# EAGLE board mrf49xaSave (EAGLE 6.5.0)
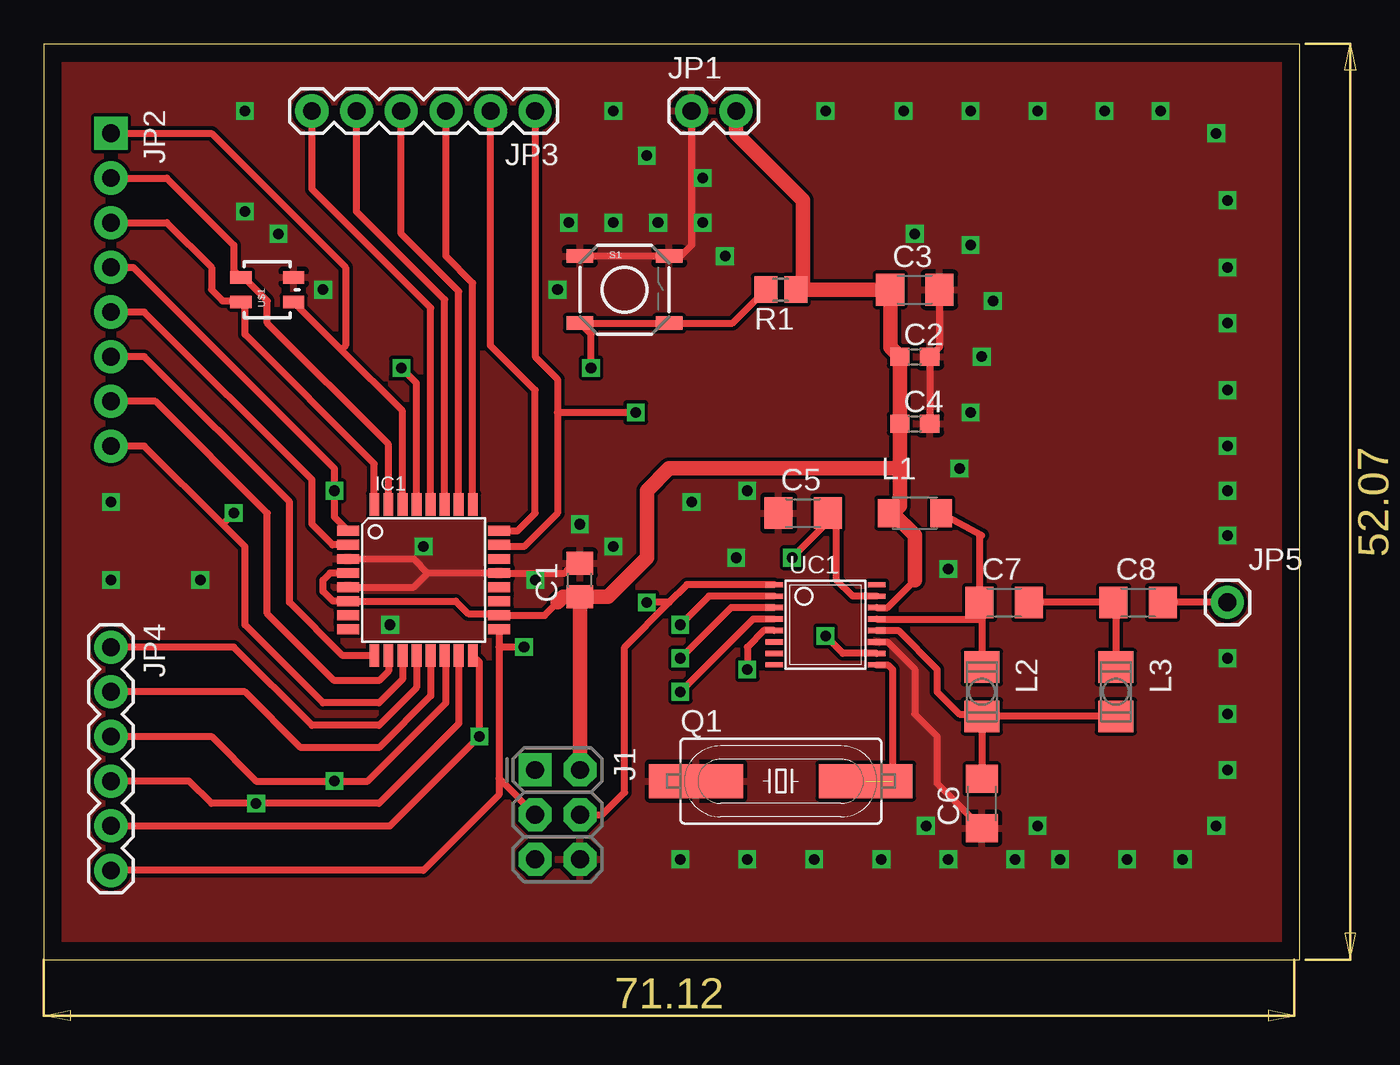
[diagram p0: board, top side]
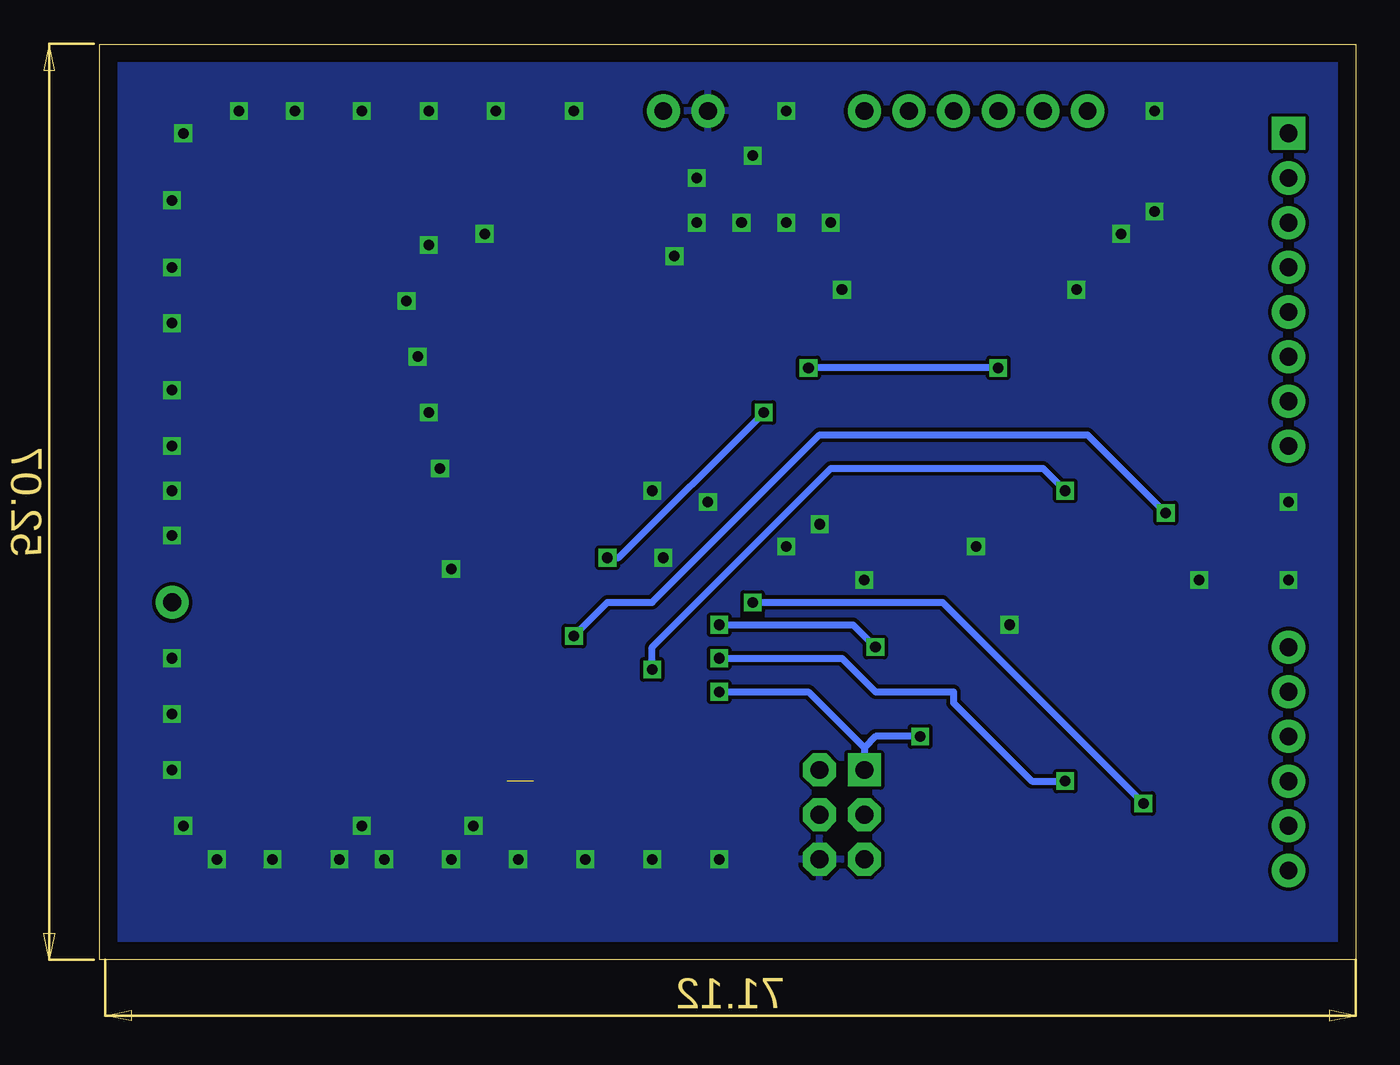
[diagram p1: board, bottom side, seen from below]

Size 74.59 x 55.55 mm. Coordinates in mm from the lower left corner, seen from the top.
Outline: 0,3.48 71.42,3.48 71.42,55.54 0,55.54 0,3.48
Copper layers (1*16): Top 0.035mm / dielectric 1.5mm / Bottom 0.035mm
Design rules "default": minimum track width 10mil, minimum drill 24mil, track to track 8mil, track to pad 8mil, pad to pad 8mil, via to via 8mil, smd to smd 8mil, copper to edge 40mil, drill to drill 8mil, minimum pad ring 10mil, minimum via ring 8mil, stop-mask expansion 4mil, vias tented up to drill 0mil, thermal gap 10mil

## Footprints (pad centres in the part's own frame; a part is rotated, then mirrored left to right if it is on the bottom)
C0805 = smd 1.3 x 1.5: 1 -0.95,0; 2 0.95,0
C0603 = smd 1.1 x 1: 1 -0.85,0; 2 0.85,0
C1206 = smd 1.6 x 1.8: 1 -1.4,0; 2 1.4,0
TQFP32-08 = smd 1.27 x 0.559: 1 -4.293,2.8; 2 -4.293,2; 3 -4.293,1.2; 4 -4.293,0.4; 5 -4.293,-0.4; 6 -4.293,-1.2; 7 -4.293,-2; 8 -4.293,-2.8; 17 4.293,-2.8; 18 4.293,-2; 19 4.293,-1.2; 20 4.293,-0.4; 21 4.293,0.4; 22 4.293,1.2; 23 4.293,2; 24 4.293,2.8 | smd 0.559 x 1.27: 9 -2.8,-4.293; 10 -2,-4.293; 11 -1.2,-4.293; 12 -0.4,-4.293; 13 0.4,-4.293; 14 1.2,-4.293; 15 2,-4.293; 16 2.8,-4.293; 25 2.8,4.293; 26 2,4.293; 27 1.2,4.293; 28 0.4,4.293; 29 -0.4,4.293; 30 -1.2,4.293; 31 -2,4.293; 32 -2.8,4.293
2X3-NS = drill 1.016 pad 1.88 square: 1 -2.54,-1.27 | drill 1.016 pad 1.88 octagon: 2 -2.54,1.27; 3 0,-1.27; 4 0,1.27; 5 2.54,-1.27; 6 2.54,1.27
1X02 = drill 1.016 pad 1.88: 1 0,0; 2 2.54,0
1X08_PIN1_NO_SILK = drill 1.016 pad 1.88 square: 1 0,0 | drill 1.016 pad 1.88: 2 2.54,0; 3 5.08,0; 4 7.62,0; 5 10.16,0; 6 12.7,0; 7 15.24,0; 8 17.78,0
1X06 = drill 1.016 pad 1.88: 1 0,0; 2 2.54,0; 3 5.08,0; 4 7.62,0; 5 10.16,0; 6 12.7,0
1X01 = drill 1.016 pad 1.88: 1 0,0
L3216C = smd 1.2 x 1.6: 1 -1.5,0; 2 1.5,0
L3225P = smd 1.8 x 2: 1 -1.4,0; 2 1.4,0
HC49UP = smd 5.334 x 1.93: 1 -4.826,0; 2 4.826,0
R2012 = smd 1.3 x 1.5: 1 -0.85,0; 2 0.85,0
TACTILE_SWITCH_SMD = smd 1.524 x 0.762: 1 -2.54,1.905; 2 2.54,1.905; 3 -2.54,-1.905; 4 2.54,-1.905
LED-TRICOLOR-SMD = smd 0.7 x 1.2: A 0.7,-1.5; B 0.7,1.5; G -0.7,1.5; R -0.7,-1.5
TSSOP16 = smd 0.305 x 0.991: 1 -2.275,-2.918; 2 -1.625,-2.918; 3 -0.975,-2.918; 4 -0.325,-2.918; 5 0.325,-2.918; 6 0.975,-2.918; 7 1.625,-2.918; 8 2.275,-2.918; 9 2.275,2.918; 10 1.625,2.918; 11 0.975,2.918; 12 0.325,2.918; 13 -0.325,2.918; 14 -0.975,2.918; 15 -1.625,2.918; 16 -2.275,2.918

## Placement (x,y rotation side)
C1  100nF  [C0805]  30.48,25.07 90 top
C2  0.01uF  [C0603]  49.53,37.77 0 top
C3  2.2uF  [C1206]  49.53,41.58 0 top
C4  47pF  [C0603]  49.53,33.95 0 top
C5  1000pF  [C1206]  43.18,28.88 0 top
C6  2.7pF  [C1206]  53.34,12.37 90 top
C7  1.2pF  [C1206]  54.61,23.79 0 top
C8  27pF  [C1206]  62.23,23.79 0 top
IC1  MEGA48/88/168-AU  [TQFP32-08]  21.59,25.07 0 top
J1  AVR_SPI_PRG_6NS  [2X3-NS]  29.21,11.73 270 top
JP1  M02PTH  [1X02]  36.83,51.73 0 top
JP2  [1X08_PIN1_NO_SILK]  3.81,50.47 270 top
JP3  [1X06]  27.94,51.73 180 top
JP4  [1X06]  3.81,21.25 270 top
JP5  M01PTH  [1X01]  67.31,23.79 0 top
L1  100nH  [L3216C]  49.53,28.88 0 top
L2  8.2nH  [L3225P]  53.34,18.71 270 top
L3  22nH  [L3225P]  60.96,18.71 270 top
Q1  10MHz  [HC49UP]  41.91,13.64 0 top
R1  10K  [R2012]  41.91,41.58 180 top
S1  [TACTILE_SWITCH_SMD]  33.02,41.58 0 top
U$1  LED-TRICOLOR  [LED-TRICOLOR-SMD]  12.7,41.58 90 top
UC1  MRF49XATSSOP163  [TSSOP16]  44.45,22.53 270 top

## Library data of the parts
C1-C8 L1-L3 = rcl
IC1 = avr-6
J1 JP1-JP5 = SparkFun-Connectors
Q1 = SparkFun
R1 = resistor
S1 = SparkFun-Electromechanical; PROD_ID: SWCH-08247
U$1 = SparkFun-LED
UC1 = nicolas

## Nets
+3V3: C1.1 C2.1 C3.1 C4.1 IC1.4 IC1.6 IC1.18 J1.2 JP1.2 L1.1 R1.1 UC1.14
BLUE: IC1.31 JP2.2 U$1.B
CS: IC1.14 JP4.3 UC1.3
GND: C1.2 C2.2 C3.2 C4.2 C5.1 C6.1 IC1.3 IC1.5 IC1.21 J1.6 JP1.1 Q1.1 S1.1 S1.2 U$1.A UC1.11
GRN: IC1.32 JP2.3 U$1.G
IRQ: IC1.1 JP2.4 UC1.5
N$1: IC1.24 JP3.2
N$2: IC1.25 JP3.3
N$3: IC1.26 JP3.4
N$4: IC1.27 JP3.5
N$5: IC1.28 JP3.6
N$9: Q1.2 UC1.9
N$10: C7.1 L1.2 L2.1 UC1.13
N$11: C7.2 C8.1 L3.1
N$12: C6.2 L2.2 L3.2 UC1.12
N$13: C8.2 JP5.1
N$16: IC1.2 JP2.5
N$17: IC1.9 JP2.6
N$18: IC1.10 JP2.7
N$20: IC1.12 JP4.1
N$21: IC1.13 JP4.2
PB7: IC1.8
RED: IC1.30 JP2.1 U$1.R
RESET_HW: J1.5
RSSI: C5.2 IC1.23 JP3.1 UC1.15
RST: IC1.11 JP2.8 UC1.10
RST_HW: IC1.29 R1.2 S1.3 S1.4
SCK: IC1.17 J1.3 JP4.6 UC1.2
SDI: IC1.15 J1.4 JP4.4 UC1.1
SDO: IC1.16 J1.1 JP4.5 UC1.4

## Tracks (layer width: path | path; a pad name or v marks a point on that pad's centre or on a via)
+3V3
  Top 0.406: 29.21,23.79 28.48,23.07 IC1.18 25.79,23.16 24.13,23.16 23.43,23.86 IC1.6 16.44,23.86 15.87,24.43 15.87,25.07 16.28,25.46 IC1.4 | UC1.14 47.96,23.5 49.53,25.07
  Top 0.813: JP1.2 39.37,50.47 43.18,46.66 43.18,42 R1.1 C3.1 48.13,38.31 C2.1 C4.1 48.68,31.42 | 48.68,31.42 48.68,29.29 48.26,28.88 | C1.1 29.53,24.11 29.21,23.79 | L1.1 48.26,28.88 | 48.26,28.88 49.53,27.61 49.53,25.07 | C1.1 32.07,24.11 34.29,26.34 34.29,30.14 35.56,31.42 48.68,31.42 | J1.2 C1.1
BLUE
  Top 0.406: JP2.2 6.99,47.93 10.79,44.11 10.79,42.68 U$1.B 11.26,42.21 11.43,42.21 12.7,40.94 12.7,39.67 19.59,32.78 IC1.31
CS  (via drill 0.6)
  Top 0.406: UC1.3 39.08,23.5 v36.19,20.62 | IC1.14 22.86,20.7 22.86,18.08 18.42,13.64 v16.51,13.64 12.07,13.64 9.53,16.18 JP4.3
  Bottom 0.406: v36.19,20.62 29.21,20.62 27.3,18.71 22.86,18.71 22.86,18.08 18.42,13.64 v16.51,13.64
GND  (via drill 0.6)
  Top 0.406: UC1.11 47.96,21.55 49.53,19.99 49.53,17.45 50.8,16.18 50.8,13.51 C6.1 | IC1.3 21.03,26.27 21.82,25.46 | 21.82,25.46 IC1.21 29.61,25.46 29.85,25.7 | IC1.5 21.03,24.67 21.82,25.46 | JP1.1 36.83,44.11 36.19,43.48 S1.1 | C3.2 50.93,38.31 C2.2 C4.2
  other vias: 11.43,51.73 32.39,51.73 44.45,51.73 37.46,47.93 34.29,49.2 38.73,43.48 37.46,45.39 34.92,45.39 32.39,45.39 29.85,45.39 29.21,41.58 48.89,51.73 52.7,51.73 56.52,51.73 60.33,51.73 63.5,51.73 66.67,50.47 67.31,46.66 67.31,42.84 67.31,39.67 67.31,35.86 67.31,32.69 67.31,30.14 67.31,27.61 67.31,20.62 67.31,17.45 67.31,14.27 66.67,11.1 64.77,9.19 61.59,9.19 57.78,9.19 56.52,11.1 50.16,11.1 55.24,9.19 51.44,9.19 47.62,9.19 43.81,9.19 40,9.19 36.19,9.19 3.81,25.07 3.81,29.51 8.89,25.07 27.94,25.07 30.48,28.24 40,30.14 36.83,29.51 39.37,26.34 32.39,26.97 49.53,44.75 52.7,44.11 53.97,40.94 53.34,37.77 52.7,34.59 52.07,31.42 11.43,46.02 13.33,44.75 15.87,41.58 51.44,25.7 21.59,26.97 19.68,22.53
  pour Top: 0,55.55 71.75,55.55 71.75,3.48 0,3.48
  pour Bottom: 0,55.55 71.75,55.55 71.75,3.48 0,3.48
GRN
  Top 0.406: JP2.3 6.99,45.39 9.53,42.84 9.53,41.58 10.16,40.94 11.14,40.94 U$1.G 11.43,40.64 11.43,39.03 18.79,31.68 IC1.32
IRQ  (via drill 0.6)
  Top 0.406: UC1.5 40.95,22.2 40,21.25 v40,19.99 | IC1.1 16.51,28.65 v16.51,30.14 16.51,31.42 5.08,42.84 JP2.4
  Bottom 0.406: v40,19.99 40,21.25 29.85,31.42 17.78,31.42 v16.51,30.14
N$1
  Top 0.406: IC1.24 26.93,27.86 27.94,28.88 27.94,35.86 25.4,38.4 JP3.2
N$2
  Top 0.406: IC1.25 24.39,41.95 22.86,43.48 JP3.3
N$3
  Top 0.406: IC1.26 23.59,41.48 20.32,44.75 JP3.4
N$4
  Top 0.406: IC1.27 22.79,41.01 17.78,46.02 JP3.5
N$5
  Top 0.406: IC1.28 21.99,40.54 15.24,47.29 JP3.6
N$9  (1 unrouted)
  Top 0.406: UC1.9 47.99,20.25 48.26,19.99 48.26,13.64
N$10
  Top 0.406: C7.1 53.34,23.79 L2.1 | L1.2 53.34,27.61 53.21,27.61 C7.1 | UC1.13 53.21,22.85 C7.1
N$11
  Top 0.406: C7.2 C8.1 60.96,23.79 L3.1
N$12
  Top 0.406: L3.2 L2.2 | L2.2 C6.2 | UC1.12 48.58,22.2 50.8,19.99 50.8,18.71 52.07,17.45 53.21,17.45 L2.2
N$13
  Top 0.406: JP5.1 C8.2
N$16
  Top 0.406: IC1.2 16.42,27.07 15.24,28.24 15.24,30.78 5.71,40.31 JP2.5
N$17
  Top 0.406: IC1.9 16.99,20.77 13.97,23.79 13.97,29.51 5.71,37.77 JP2.6
N$18
  Top 0.406: IC1.10 19.59,19.89 19.05,19.35 16.51,19.35 12.7,23.16 12.7,28.88 6.35,35.23 JP2.7
N$20
  Top 0.406: IC1.12 21.19,18.95 19.05,16.81 15.24,16.81 10.79,21.25 JP4.1
N$21
  Top 0.406: IC1.13 21.99,18.48 19.05,15.54 14.61,15.54 11.43,18.71 JP4.2
RED
  Top 0.406: IC1.30 20.39,34.69 16.91,38.17 | 16.91,38.17 U$1.R | JP2.1 9.53,50.47 17.14,42.84 17.14,38.4 16.91,38.17
RSSI  (via drill 0.6)
  Top 0.406: UC1.15 46,24.15 45.08,25.07 45.08,28.88 C5.2 44.58,28.37 v42.55,26.34 | v33.66,34.59 29.21,34.59 | 29.21,34.59 29.21,28.88 27.3,26.97 25.98,26.97 IC1.23 | JP3.1 27.94,37.77 29.21,36.5 29.21,34.59
  Bottom 0.406: v42.55,26.34 41.91,26.34 v33.66,34.59
RST  (via drill 0.6)
  Top 0.406: IC1.11 20.39,19.42 19.05,18.08 15.87,18.08 11.43,22.53 11.43,26.97 10.16,28.24 | JP2.8 5.71,32.69 10.16,28.24 | UC1.10 45.44,20.9 v44.45,21.89 | v10.79,28.88 10.16,28.24
  Bottom 0.406: v44.45,21.89 42.55,23.79 40,23.79 30.48,33.32 15.24,33.32 v10.79,28.88
RST_HW  (via drill 0.6)
  Top 0.406: R1.2 39.16,39.67 S1.4 S1.3 31.11,39.03 v31.11,37.13 | IC1.29 21.19,36.26 v20.32,37.13
  Bottom 0.406: v20.32,37.13 v31.11,37.13
SCK  (via drill 0.6)
  Top 0.406: IC1.17 25.88,21.25 | 25.88,21.25 25.88,13.79 | JP4.6 21.59,8.56 25.88,12.85 25.88,13.79 | UC1.2 37.82,24.15 v36.19,22.53 | v27.3,21.25 25.88,21.25 | 25.88,13.79 J1.3
  Bottom 0.406: v36.19,22.53 28.57,22.53 v27.3,21.25
SDI  (via drill 0.6)
  Top 0.406: J1.4 31.75,11.73 33.02,13 33.02,21.25 35.56,23.79 | 35.56,23.79 36.56,24.8 UC1.1 | 35.56,23.79 v34.29,23.79 | JP4.4 8.25,13.64 9.53,12.37 v12.07,12.37 19.05,12.37 23.59,16.91 IC1.15
  Bottom 0.406: v34.29,23.79 23.5,23.79 v12.07,12.37
SDO  (via drill 0.6)
  Top 0.406: UC1.4 40.33,22.85 v36.19,18.71 | IC1.16 24.76,20.4 v24.76,16.18 19.68,11.1 JP4.5
  Bottom 0.406: v36.19,18.71 31.11,18.71 27.94,15.54 | 27.94,15.54 J1.1 | v24.76,16.18 27.3,16.18 27.94,15.54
